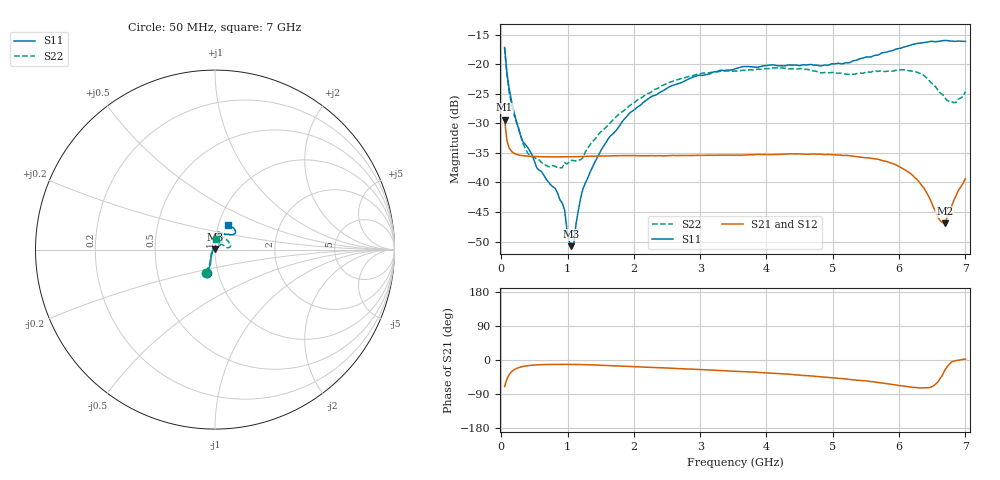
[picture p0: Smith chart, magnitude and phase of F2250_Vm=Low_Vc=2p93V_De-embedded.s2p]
! Integrated Device Technology
! Corporate Headquarters
! 6024 Silver Creek Valley Road
! San Jose, CA 95138  USA
! Phone:  1-408-284-8200
! Toll Free:  1-800-223-1366
! Webpage:  http://www.idt.com/
! Timing and RF Division
! 515 Groton Road, Suite 102
! Westford, MA 01886-6024
! Device:  F2250
! Description: Voltage Variable RF Attenuator
! Frequency:  50.0 -  6000.00 MHz
! Package:  3x3 mm Thin QFN Plastic Package: 16 pin
! Ports:  2 RF, 3 DC
!  Pin  1  = GND
!  Pin  2  = NC
!  Pin  3  = RF1  = Port 1
!  Pin  4  = NC
!  Pin  5  = GND
!  Pin  6  = GND
!  Pin  7  = GND
!  Pin  8  = GND
!  Pin  9  = NC
!  Pin 10  = RF2  = Port 2
!  Pin 11  = NC
!  Pin 12  = GND
!  Pin 13  = GND
!  Pin 14  = VCNTRL
!  Pin 15  = VDD
!  Pin 16  = VMODE
! Vcntrl:  2.930 Volts
! Vmode:  +0.000 Volts
! Vdd:  +3.30  Volts
! Current:  1.176 mA
! Data:  The device was measured on a the F2250 evaluation board which has
!  individual transmission lines to the RF pins.  Data was collected
!  using a calibrated network analyzer.  The evaluation board was
!  de-embedded using a TRL calibration technique.
!  The reference plane is the edge of the package pin.
! Misc:  SN 10
!  Action Tracker AT0258
! Date Measured:  2014-11-26
! Date:  2015-10-15  MJV
! Note:
!  Integrated Device Technology supplies this data as a sample of measured
!  data at the package pin for this product.  Your particular data for this
!  product may vary.
!  Data was taken at 25 degrees C.
!  Integrated Device Technology reserves the right to change this data at anytime.
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# GHz S dB R 50
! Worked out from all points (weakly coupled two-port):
!   201 points, 50 MHz to 7 GHz, reference 50 ohm
!   highest |S21| = -29.42 dB at 50 MHz (marker M1); lowest = -46.9 dB at 6.687 GHz (marker M2)
!   lowest |S11| = -50.8 dB at 1.058 GHz (marker M3), VSWR 1.01, Z = 49.8 + j0.239 ohm
!   |S11| at or under -10 dB: start of sweep to end of sweep
!   |S22| runs from -37.5 to -17.3 dB; largest |S21 - S12| = 7.2e-05
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0.05  -17.18 -108.6  -29.42 -69.8  -29.41 -69.8  -17.28 -111.0
0.08475  -21.45 -107.4  -32.92 -50.4  -32.92 -50.3  -21.74 -110.2
0.15425  -26.23 -116.6  -34.76 -31.1  -34.76 -31.1  -26.81 -122.5
0.29325  -32.22 -127.9  -35.43 -18.5  -35.43 -18.5  -32.09 -137.4
0.3975  -34.09 -141.8  -35.56 -15.0  -35.56 -15.0  -35.03 -160.5
0.91875  -43.49 158.0  -35.69 -11.5  -35.69 -11.5  -37.53 133.4
0.9535  -44.60 170.1  -35.68 -11.5  -35.69 -11.5  -36.65 131.0
1.023  -49.94 142.8  -35.68 -11.6  -35.67 -11.6  -36.62 115.8
1.05775  -50.78 124.0  -35.67 -11.6  -35.67 -11.6  -36.28 110.7
1.0925  -50.49 89.6  -35.66 -11.7  -35.65 -11.7  -36.30 106.3
1.12725  -47.01 66.5  -35.65 -11.8  -35.65 -11.8  -36.38 100.5
1.2315  -41.08 44.4  -35.61 -12.1  -35.61 -12.1  -35.80 85.8
1.6485  -32.11 42.1  -35.52 -14.6  -35.52 -14.7  -29.87 64.5
1.96125  -28.04 42.3  -35.46 -17.2  -35.46 -17.2  -26.80 56.8
2.37825  -24.87 47.3  -35.48 -20.3  -35.48 -20.3  -23.99 56.8
3.525  -20.79 72.5  -35.40 -29.5  -35.40 -29.5  -21.19 74.7
4.7065  -20.17 72.3  -35.19 -42.6  -35.19 -42.7  -21.14 72.2
5.85325  -17.81 40.4  -36.63 -63.4  -36.63 -63.5  -21.14 23.1
6.27025  -16.50 40.0  -39.50 -72.8  -39.51 -72.9  -21.37 9.7
6.68725  -15.99 48.7  -46.89 -27.7  -46.88 -27.2  -25.64 28.6
6.861  -16.14 55.1  -42.20 -1.4  -42.16 -1.4  -26.44 58.0
7  -16.13 63.2  -39.38 1.9  -39.33 1.7  -24.64 83.1
